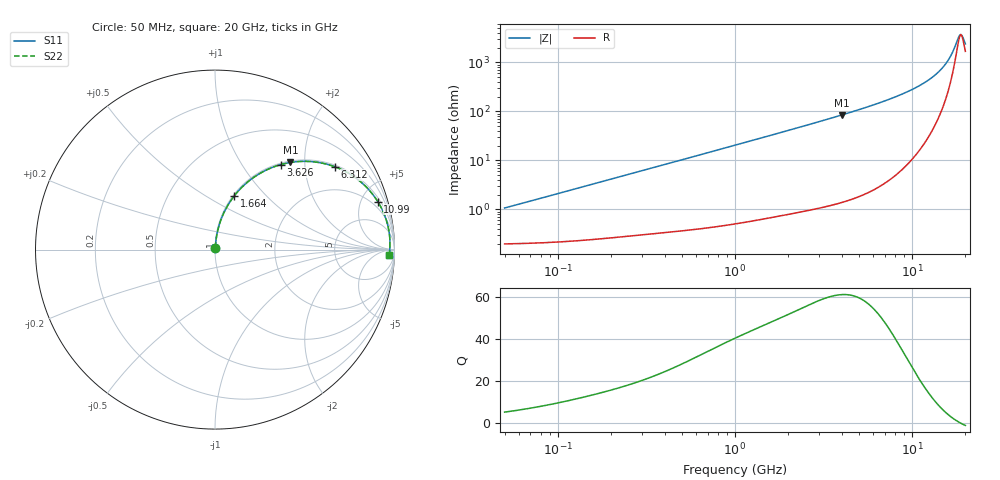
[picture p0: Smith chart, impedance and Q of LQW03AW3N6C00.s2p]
!Murata Part Number: LQW03AW3N6C00
!These Parameters are Measured in Series Mode Connection
!  o--[Z]--o
!Port1  Port2
!  o-------o
!Freq. Start=50[MHz] Stop=20[GHz], 401[Steps]
# Hz S RI R 50
!Freq.(Hz) S11(Real) S11(Imag) S21(Real) S21(Imag) S12(Real) S12(Imag) S22(Real) S22(Imag)
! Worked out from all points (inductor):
!   401 points, 50 MHz to 20 GHz, reference 50 ohm
!   read as one part in series: L = 3.34 nH near 51.52 MHz
!   highest Q = 61 at 4.027 GHz (marker M1), where L = 3.35 nH
!   self-resonance near 18.9 GHz
!   S11 on the Smith chart (normalised r, x): 50 MHz: 1.00, +0.02; 1.664 GHz: 1.01, +0.68; 3.626 GHz: 1.03, +1.52; 6.312 GHz: 1.05, +2.85; 10.99 GHz: 1.32, +6.66; 20 GHz: 35, -34
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5e7  0.00209 0.0105  0.9979 -0.0105  0.9979 -0.0105  0.00209 0.0105
1.364002e8  0.00313 0.0283  0.9969 -0.0283  0.9969 -0.0283  0.00313 0.0283
3.721004e8  0.00904 0.0756  0.991 -0.0756  0.991 -0.0756  0.00904 0.0756
6.285508e8  0.0201 0.1255  0.9799 -0.1255  0.9799 -0.1255  0.0201 0.1255
1e9  0.0444 0.194  0.9556 -0.194  0.9556 -0.194  0.0444 0.194
1.664083e9  0.1084 0.3007  0.8916 -0.3007  0.8916 -0.3007  0.1084 0.3007
2.728004e9  0.2438 0.4207  0.7562 -0.4207  0.7562 -0.4207  0.2438 0.4207
3.626126e9  0.367 0.4738  0.633 -0.4738  0.633 -0.4738  0.367 0.4738
4.026975e9  0.4201 0.4854  0.5799 -0.4854  0.5799 -0.4854  0.4201 0.4854
5.041459e9  0.5428 0.4898  0.4572 -0.4898  0.4572 -0.4898  0.5428 0.4898
6.311513e9  0.6678 0.4616  0.3322 -0.4616  0.3322 -0.4616  0.6678 0.4616
7.442007e9  0.7531 0.4201  0.2469 -0.4201  0.2469 -0.4201  0.7531 0.4201
9.178299e9  0.8458 0.3458  0.1542 -0.3458  0.1542 -0.3458  0.8458 0.3458
1.098561e10  0.9068 0.2678  0.0932 -0.2678  0.0932 -0.2678  0.9068 0.2678
1.314879e10  0.9486 0.1817  0.0514 -0.1817  0.0514 -0.1817  0.9486 0.1817
1.504638e10  0.9671 0.1144  0.0329 -0.1144  0.0329 -0.1144  0.9671 0.1144
1.646126e10  0.9734 0.0691  0.0266 -0.0691  0.0266 -0.0691  0.9734 0.0691
1.721783e10  0.9747 0.0465  0.0253 -0.0465  0.0253 -0.0465  0.9747 0.0465
1.800918e10  0.9748 0.0239  0.0252 -0.0239  0.0252 -0.0239  0.9748 0.0239
1.855685e10  0.9742 0.00895  0.0258 -0.00895  0.0258 -0.00895  0.9742 0.00895
1.912117e10  0.9731 -0.00594  0.0269 0.00594  0.0269 0.00594  0.9731 -0.00594
2e10  0.9705 -0.0281  0.0295 0.0281  0.0295 0.0281  0.9705 -0.0281
